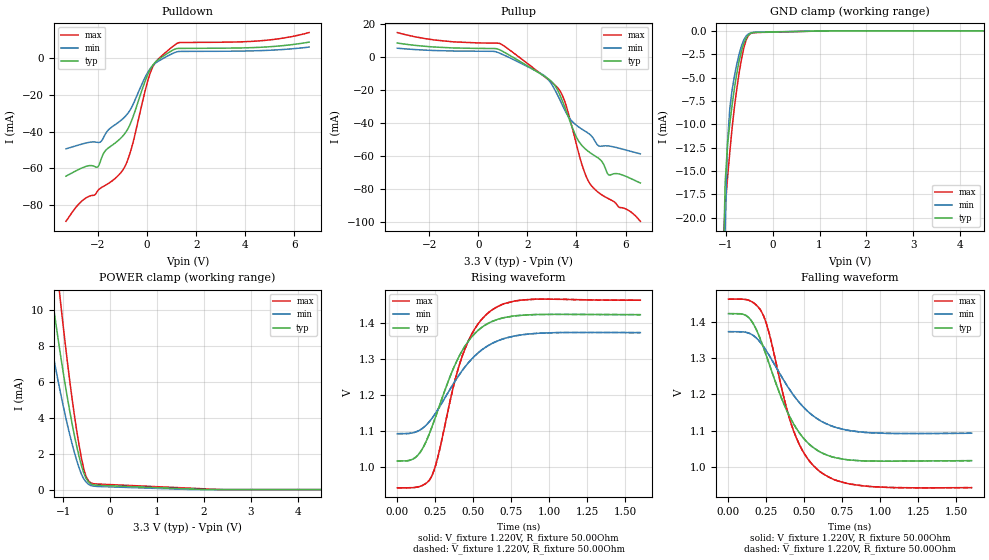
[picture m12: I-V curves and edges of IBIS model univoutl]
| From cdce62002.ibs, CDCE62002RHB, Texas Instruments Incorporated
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|   Model   univoutl
[Model]   univoutl
Model_type   3-state
Polarity   Non-Inverting
Cref   =   0.00
Rref   =   50
|Variable   typ   min   max
C_comp   1.488e-12   1.482e-12   1.523e-12
[Model Spec]
Vref   1.25V   1.15V   1.375V
Vmeas   1.25V   1.15V   1.375V
|Variable   typ   min   max
[Voltage range]   3.3   3.0   3.6
|Variable   typ   min   max
[Temperature range]  40   100   -40
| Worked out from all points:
|   slope of the pulldown table from 0 to 0.495 V, typ, clamps not added: 52.5 ohm
|   slope of the pullup table from 0 to 0.495 V, typ, clamps not added: 10.8 kohm
|   GND clamp passes 1 mA (typ) near -0.58 V on its own axis
|   POWER clamp passes 1 mA (typ) near -0.57 V on its own axis
|   falling waveform, V_fixture 1.220V, R_fixture 50.00Ohm: 20-80 % time 240ps typ, 280ps min, 211ps max; typ from 1.42 V to 1.02 V
|   rising waveform, V_fixture 1.220V, R_fixture 50.00Ohm: 20-80 % time 239ps typ, 282ps min, 200ps max; typ from 1.02 V to 1.42 V
|   rising waveform, V_fixture 1.220V, R_fixture 50.00Ohm: 20-80 % time 239ps typ, 282ps min, 200ps max; typ from 1.02 V to 1.42 V
|   falling waveform, V_fixture 1.220V, R_fixture 50.00Ohm: 20-80 % time 240ps typ, 280ps min, 211ps max; typ from 1.42 V to 1.02 V
[Pulldown]
|   Voltage   I(typ)   I(min)   I(max)
-3.3V     -64.32mA   -49.44mA   -88.92mA
-2.703V   -60.19mA   -47.03mA   -78.49mA
-2.007V   -59.31mA   -45.92mA   -72.26mA
-1.708V   -50.67mA   -41.67mA   -69.4mA
-961.8mV  -42.07mA   -32.76mA   -60.51mA
-613.6mV  -33.57mA   -26.49mA   -48.17mA
-66.33mV  -12.2mA    -10.21mA   -17.29mA
182.4mV   -4.943mA   -4.832mA   -6.331mA
431.2mV   -1.132mA   -1.934mA   -901.9uA
1.078V    4.53mA     2.728mA    6.643mA
4.909V    6.12mA     4.227mA    9.792mA
6.6V      8.704mA    6.006mA    13.92mA
[GND Clamp]
|   Voltage   I(typ)   I(min)   I(max)
-3.3V     -4.022A    -3.907A    -4.266A
-1.061V   -27.23mA   -43.89mA   -23.06mA
-1.012V   -16.24mA   -21.24mA   -18.95mA
-961.8mV  -12.25mA   -11.96mA   -15.82mA
-912.1mV  -9.874mA   -8.274mA   -12.94mA
-862.3mV  -7.89mA    -6.288mA   -10.34mA
-762.8mV  -4.522mA   -3.552mA   -6.176mA
-663.3mV  -2.151mA   -1.601mA   -3.015mA
-563.8mV  -779.3uA   -554.1uA   -972.9uA
-464.3mV  -264.9uA   -209.2uA   -276uA
1.227V    0A         -449.7nA   0A
6.6V      0A         0A         0A
[Pullup]
|   Voltage   I(typ)   I(min)   I(max)
-3.3V     8.704mA    5.566mA    15.07mA
878.9mV   4.518mA    2.501mA    8.413mA
2.521V    -9.902mA   -9.588mA   -9.69mA
3.068V    -16.07mA   -18.35mA   -16.17mA
3.416V    -26.18mA   -28.72mA   -22.91mA
4.013V    -48.96mA   -41.51mA   -53.82mA
4.312V    -55.01mA   -44.53mA   -69.18mA
4.56V     -58.06mA   -47.08mA   -77.11mA
4.909V    -61.49mA   -53.91mA   -82.32mA
5.307V    -71.46mA   -53.89mA   -85.99mA
5.754V    -71.01mA   -55.33mA   -91.31mA
6.6V      -76.42mA   -58.67mA   -99.7mA
[POWER Clamp]
|   Voltage   I(typ)   I(min)   I(max)
-3.3V     434.9mA    385mA      510.3mA
-1.459V   15.25mA    11.2mA     21.25mA
-1.41V    14.21mA    10.41mA    19.82mA
-1.26V    11.23mA    8.169mA    15.68mA
-1.211V   10.27mA    7.457mA    14.36mA
-1.061V   7.576mA    5.441mA    10.58mA
-862.3mV  4.403mA    3.086mA    6.102mA
-663.3mV  1.864mA    1.229mA    2.504mA
-514.1mV  630uA      424.6uA    736.8uA
-414.6mV  324.6uA    230.2uA    378.2uA
2.371V    0A         0A         2.594uA
6.6V      0A         0A         0A
[Ramp]
R_load = 50.00Ohm
|   typ   min   max
dV/dt_r   243.237mV/238.776ps 168.023mV/281.936ps 311.885mV/199.972ps
dV/dt_f   243.237mV/239.793ps 168.023mV/279.558ps 311.885mV/211.102ps
[Falling Waveform]
V_fixture = 1.220V
V_fixture_min = 1.232V
V_fixture_max = 1.200V
R_fixture = 50.00Ohm
|   Time   V(typ)   V(min)   V(max)
0s        1.422V     1.373V     1.462V
130ps     1.413V     1.369V     1.46V
220ps     1.34V      1.338V     1.425V
266ps     1.286V     1.308V     1.371V
372ps     1.166V     1.233V     1.178V
428ps     1.119V     1.198V     1.1V
503ps     1.074V     1.16V      1.034V
603ps     1.041V     1.128V     986.5mV
897ps     1.016V     1.095V     946.9mV
1.6ns     1.017V     1.092V     942.4mV
[Rising Waveform]
V_fixture = 1.220V
V_fixture_min = 1.232V
V_fixture_max = 1.200V
R_fixture = 50.00Ohm
|   Time   V(typ)   V(min)   V(max)
0s        1.017V     1.092V     942.4mV
128ps     1.03V      1.098V     944.3mV
223ps     1.105V     1.132V     971.5mV
265ps     1.154V     1.158V     1.024V
370ps     1.274V     1.231V     1.223V
429ps     1.324V     1.268V     1.309V
508ps     1.369V     1.307V     1.381V
610ps     1.401V     1.339V     1.431V
826ps     1.421V     1.367V     1.463V
1.6ns     1.422V     1.373V     1.462V
[Rising Waveform]
V_fixture = 1.220V
V_fixture_min = 1.232V
V_fixture_max = 1.200V
R_fixture = 50.00Ohm
|   Time   V(typ)   V(min)   V(max)
0s        1.017V     1.092V     942.4mV
128ps     1.03V      1.098V     944.3mV
223ps     1.105V     1.132V     971.5mV
265ps     1.154V     1.158V     1.024V
370ps     1.274V     1.231V     1.223V
429ps     1.324V     1.268V     1.309V
508ps     1.369V     1.307V     1.381V
610ps     1.401V     1.339V     1.431V
826ps     1.421V     1.367V     1.463V
1.6ns     1.422V     1.373V     1.462V
[Falling Waveform]
V_fixture = 1.220V
V_fixture_min = 1.232V
V_fixture_max = 1.200V
R_fixture = 50.00Ohm
|   Time   V(typ)   V(min)   V(max)
0s        1.422V     1.373V     1.462V
130ps     1.413V     1.369V     1.46V
220ps     1.34V      1.338V     1.425V
266ps     1.286V     1.308V     1.371V
372ps     1.166V     1.233V     1.178V
428ps     1.119V     1.198V     1.1V
503ps     1.074V     1.16V      1.034V
603ps     1.041V     1.128V     986.5mV
897ps     1.016V     1.095V     946.9mV
1.6ns     1.017V     1.092V     942.4mV
